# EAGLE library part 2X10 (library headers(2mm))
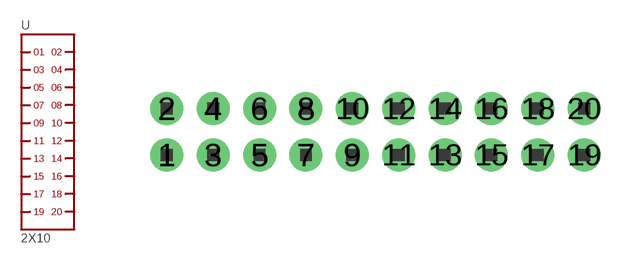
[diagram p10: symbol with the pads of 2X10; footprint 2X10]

Designator prefix -

## 2X10  [2X10]
1  1
2  2
3  3
4  4
5  5
6  6
7  7
8  8
9  9
10  10
11  11
12  12
13  13
14  14
15  15
16  16
17  17
18  18
19  19
20  20

## Footprint 2X10 (pad centres in mm)
drill 0.8 pad 1.422: 1 -9,-1; 2 -9,1; 3 -7,-1; 4 -7,1; 5 -5,-1; 6 -5,1; 7 -3,-1; 8 -3,1; 9 -1,-1; 10 -1,1; 11 1,-1; 12 1,1; 13 3,-1; 14 3,1; 15 5,-1; 16 5,1; 17 7,-1; 18 7,1; 19 9,-1; 20 9,1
